TYPE STR_EL2889 :
STRUCT
	Out_Bit0		:	BOOL	;
	Out_Bit1		:	BOOL	;
	Out_Bit2		:	BOOL	;
	Out_Bit3		:	BOOL	;
	Out_Bit4		:	BOOL	;
	Out_Bit5		:	BOOL	;
	Out_Bit6		:	BOOL	;
	Out_Bit7		:	BOOL	;
	Out_Bit8		:	BOOL	;
	Out_Bit9		:	BOOL	;
	Out_Bit10		:	BOOL	;
	Out_Bit11		:	BOOL	;
	Out_Bit12		:	BOOL	;
	Out_Bit13		:	BOOL	;
	Out_Bit14		:	BOOL	;
	Out_Bit15		:	BOOL	;

END_STRUCT
END_TYPE
